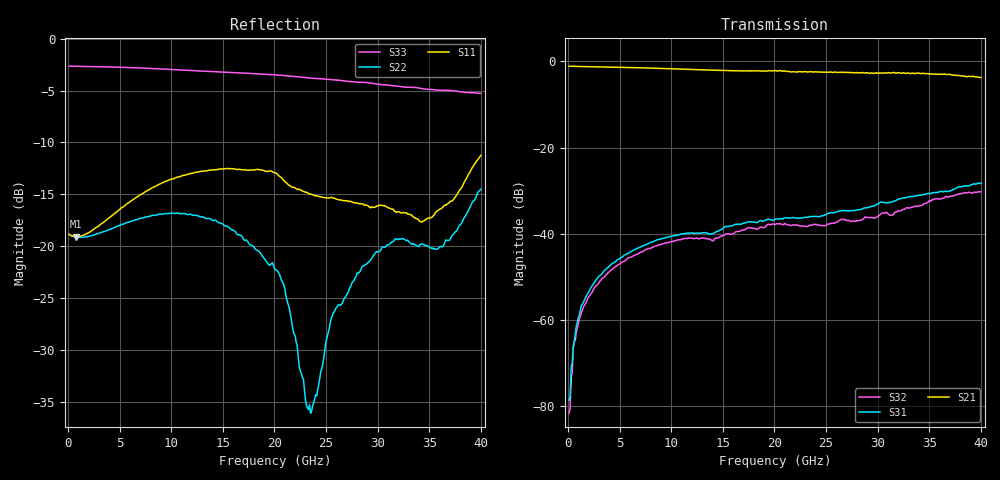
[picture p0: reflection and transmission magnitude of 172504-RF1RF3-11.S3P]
!  3-Port S-parameters saved by WinCal
! VAR MeasName=S-Parameters (CALIBRATED_DATA) read from VNA (N5245A)
! VAR MeasDate=2017-3-15 11:07:56
! VAR NAME=172504-RF1RF3-11
! VAR FILENAME=172504-RF1RF3-11.S3P
! VAR DATE=2017-3-15 11:07:56
! VAR PHYS_PORTS=1,2,3
# Hz S DB R 50
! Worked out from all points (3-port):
!   400 points, 100 MHz to 40 GHz, reference 50 ohm
!   strongest paths, dB at 100 MHz, 10.1 GHz, 20.1 GHz, 30.1 GHz, 40 GHz:
!     S21: -1.1, -1.7, -2.1, -2.7, -3.7
!     S31: -78.6, -40.5, -36.6, -32.9, -28.2
!     S32: -81.6, -41.8, -37.8, -35.8, -30.2
!   lowest |S11| = -19.1 dB at 800 MHz (marker M1), VSWR 1.25, Z = 61.9 - j3.69 ohm
!   |S11| at or under -10 dB: start of sweep to end of sweep
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1e8  -18.86 -2.6  -1.10 -0.7  -87.68 35.8
     -1.10 -0.7  -18.85 -2.4  -80.17 136.3
     -78.58 66.0  -81.59 172.9  -2.64 179.8
5e8  -19.04 -10.2  -1.13 -3.3  -66.81 112.9
     -1.13 -3.3  -19.07 -8.7  -68.17 107.0
     -66.07 101.5  -66.50 105.1  -2.64 178.9
8e8  -19.08 -15.4  -1.16 -5.1  -61.16 98.1
     -1.15 -5.1  -19.13 -13.1  -62.72 96.4
     -61.35 96.4  -62.75 98.5  -2.64 178.3
2.6e9  -18.29 -42.4  -1.24 -15.7  -51.04 77.0
       -1.24 -15.7  -18.90 -37.2  -52.34 74.4
       -51.03 75.9  -52.27 74.5  -2.68 174.7
5.8e9  -15.84 -77.6  -1.38 -34.4  -44.47 55.9
       -1.40 -34.4  -17.70 -74.7  -45.64 49.3
       -44.56 55.8  -45.60 50.3  -2.76 168.3
2.01e10  -12.92 -157.2  -2.17 -114.8  -36.30 -19.9
         -2.10 -114.8  -22.26 173.5  -37.33 -40.8
         -36.55 -18.8  -37.78 -41.0  -3.47 138.5
2.35e10  -14.98 -163.1  -2.45 -134.0  -35.95 -37.9
         -2.39 -134.0  -36.13 59.9  -37.85 -61.7
         -35.98 -36.1  -37.97 -59.8  -3.79 130.0
2.85e10  -15.94 -175.8  -2.75 -164.0  -34.08 -61.2
         -2.57 -163.6  -21.94 -47.5  -36.47 -80.6
         -34.23 -58.8  -36.66 -79.7  -4.20 117.2
3.43e10  -17.65 122.4  -2.86 157.8  -30.86 -99.8
         -2.78 158.2  -19.77 -64.5  -33.44 -114.1
         -30.92 -97.4  -33.36 -110.6  -4.81 100.5
4e10  -11.24 31.2  -3.77 117.5  -27.95 -141.4
      -3.71 115.6  -14.49 -41.9  -30.08 -160.4
      -28.19 -140.1  -30.21 -159.7  -5.26 82.6
